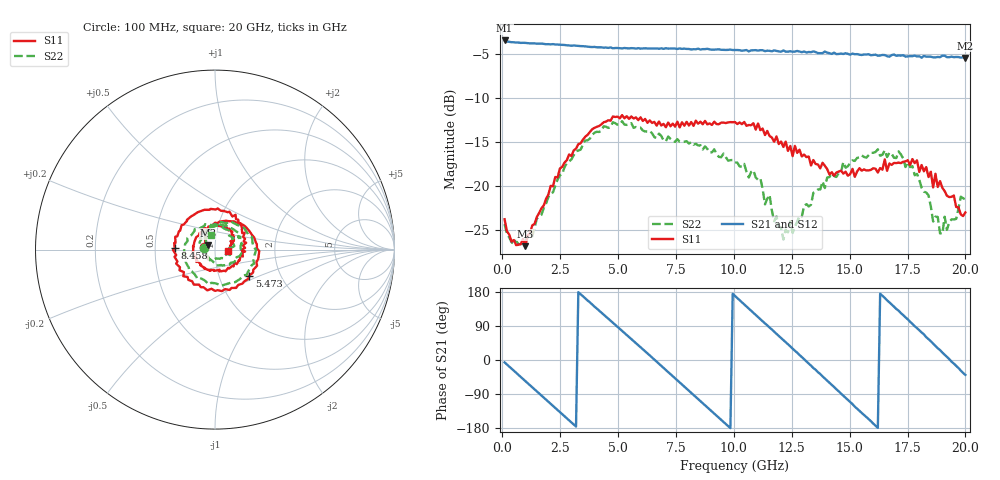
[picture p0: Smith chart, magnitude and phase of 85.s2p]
!Agilent Technologies,N5230C,MY49001569,A.09.33.09
!Agilent N5230C: A.09.33.09
!Date: Tuesday, July 28, 2015 10:10:32
!Correction: S11(Full 2 Port(1,2))
!S21(Full 2 Port(1,2))
!S12(Full 2 Port(1,2))
!S22(Full 2 Port(1,2))
!S2P File: Measurements: S11, S21, S12, S22:
# Hz S  dB  R 50
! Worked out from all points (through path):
!   201 points, 100 MHz to 20 GHz, reference 50 ohm
!   highest |S21| = -3.51 dB at 100 MHz (marker M1); lowest = -5.5 dB at 20 GHz (marker M2)
!   group delay of S21, straight-line fit = 155 ps
!   lowest |S11| = -26.9 dB at 995.5 MHz (marker M3), VSWR 1.09, Z = 46.2 + j2.14 ohm
!   |S11| at or under -10 dB: start of sweep to end of sweep
!   |S22| runs from -26.8 to -12.7 dB; largest |S21 - S12| = 0.016
!   S11 on the Smith chart (normalised r, x): 100 MHz: 0.88, +0.02; 5.473 GHz: 1.39, -0.43; 8.458 GHz: 0.63, +0.01; 20 GHz: 1.15, -0.02
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1e8  -23.84 168.2  -3.51 -6.3  -3.55 -6.0  -24.40 169.3
9.955e8  -26.89 149.2  -3.79 -55.6  -3.81 -55.7  -26.45 148.9
2.09e9  -20.04 123.8  -3.95 -115.9  -3.95 -116.1  -20.92 128.5
3.483e9  -14.78 59.6  -4.16 168.2  -4.21 167.9  -15.34 63.0
4.478e9  -12.74 10.2  -4.31 114.4  -4.31 114.2  -13.31 16.2
5.473e9  -12.43 -37.2  -4.42 60.5  -4.39 60.8  -13.08 -35.0
6.7665e9  -12.73 -100.6  -4.46 -9.8  -4.44 -10.3  -14.11 -100.7
7.662e9  -13.39 -144.1  -4.41 -59.2  -4.46 -59.5  -15.04 -145.7
8.458e9  -12.97 177.8  -4.44 -103.2  -4.55 -103.3  -15.44 173.1
9.3535e9  -13.03 134.3  -4.51 -152.4  -4.49 -152.8  -16.74 123.7
1.005e10  -12.79 105.1  -4.60 169.0  -4.68 168.9  -17.37 80.0
1.09455e10  -13.64 62.3  -4.61 119.0  -4.69 119.3  -19.09 31.0
1.17415e10  -15.03 31.1  -4.63 74.6  -4.82 74.8  -24.06 -35.9
1.2637e10  -15.49 -3.8  -4.78 24.4  -4.76 24.3  -24.68 -138.1
1.3433e10  -17.11 -42.1  -4.75 -21.1  -4.84 -21.2  -20.83 165.8
1.4826e10  -18.43 -133.7  -4.96 -99.5  -5.03 -100.3  -17.97 98.3
1.5821e10  -18.27 162.2  -5.08 -155.9  -5.17 -156.7  -16.56 55.6
1.67165e10  -17.49 106.0  -5.36 152.2  -5.21 152.4  -16.26 12.3
1.7413e10  -17.26 62.2  -5.35 112.6  -5.21 111.6  -17.90 -19.5
1.8209e10  -18.38 35.9  -5.27 67.4  -5.33 66.0  -20.70 -68.4
1.91045e10  -20.64 15.6  -5.24 13.9  -5.47 13.3  -23.54 -166.1
2e10  -23.06 -7.0  -5.50 -39.4  -5.39 -39.2  -21.58 107.1
